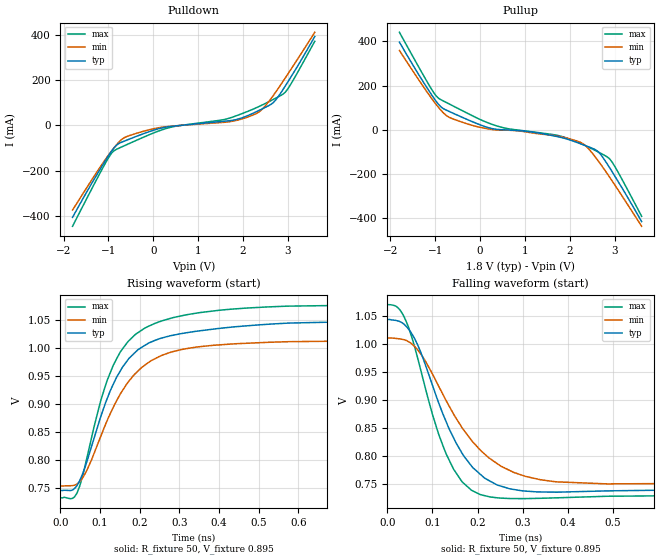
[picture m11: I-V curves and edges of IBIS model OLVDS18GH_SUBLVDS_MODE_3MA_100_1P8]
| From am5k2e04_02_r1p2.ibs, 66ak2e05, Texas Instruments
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|   Model Cell ilvds18gv
|   Model Cell olvds18gh
|   Model Cell OLVDS18GH_SUBLVDS_MODE_3MA_100_1P8
|OLVDS18GH_SUBLVDS_MODE_3MA_100_1P8
|olvds18gh.ibs [30Dec11 revision 1.0]
[Model]   OLVDS18GH_SUBLVDS_MODE_3MA_100_1P8
Model_type   Output
Polarity   Non-Inverting
Cref =  15.0001pF
Rref =  101.0000M
Vref =  0V
Vmeas =  1.08V
C_comp   1p   1p   1p
[Temperature Range]   25   125   -40
[Voltage Range]   1.8   1.62   1.98
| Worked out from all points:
|   slope of the pulldown table from 0 to 0.27 V, typ, clamps not added: 20.1 ohm
|   slope of the pullup table from 0 to 0.27 V, typ, clamps not added: 15.8 ohm
|   rising waveform, R_fixture 50, V_fixture 0.895: 20-80 % time 107ps typ, 116ps min, 96.1ps max; typ from 0.746 V to 1.04 V
|   falling waveform, R_fixture 50, V_fixture 0.895: 20-80 % time 90.7ps typ, 122ps min, 74.5ps max; typ from 1.04 V to 0.746 V
| Nom Voltages:
[Pulldown]
|   voltage   I(typ)   I(min)   I(max)
-1.8V     -406.9mA   -374.8mA   -446.6mA
-1.091V   -163.1mA   -157mA     -175.2mA
-872.7mV  -98.45mA   -98.29mA   -111.4mA
-654.5mV  -69.92mA   -54.94mA   -90.55mA
-54.55mV  -24.92mA   -17.11mA   -38.02mA
436.4mV   -3.309mA   -2.683mA   -5.734mA
1.745V    22.29mA    18.18mA    35.67mA
2.345V    65.48mA    58.17mA    83mA
2.673V    100.7mA    132mA      115.1mA
2.945V    175.7mA    211.4mA    148mA
3.109V    227.8mA    260.9mA    197.5mA
3.6V      394mA      412.8mA    372.8mA
[Pullup]
|   voltage   I(typ)   I(min)   I(max)
-1.8V     396.8mA    358.7mA    441.5mA
-1.145V   177.4mA    159.4mA    204.2mA
-927.3mV  114.3mA    100.5mA    142.1mA
-709.1mV  84.19mA    58.01mA    118.4mA
-109.1mV  30.59mA    15.72mA    56.53mA
490.9mV   -510.8uA   -2.408mA   10.05mA
1.745V    -32.6mA    -29.99mA   -26.98mA
2.291V    -68.08mA   -63.41mA   -67.31mA
2.618V    -97.7mA    -138mA     -99.79mA
2.891V    -174.1mA   -216.9mA   -133.5mA
3.109V    -246.4mA   -283.9mA   -205.6mA
3.6V      -417mA     -438.3mA   -393mA
[Ramp]
| variable   typ   min   max
dV/dt_f   9.252m/0.88253716n   5.154m/0.88425176n   11.244m/2.8474831n
dV/dt_r   4.506m/0.885501n   5.568m/3.3979628n   12.558m/4.1930989n
R_load = 50
[Rising Waveform]
R_fixture = 50
V_fixture = 0.895
V_fixture_min = 0.8825
V_fixture_max = 0.90115
|   time   V(typ)   V(min)   V(max)
0s        746.2mV    754.1mV    733.1mV
41.6ps    754.8mV    757.8mV    741.3mV
65.3ps    794.7mV    780.4mV    799.6mV
104ps     883mV      847.2mV    912.3mV
148.4ps   956.8mV    915.3mV    990.6mV
194.2ps   996.6mV    958.6mV    1.027V
238.6ps   1.014V     981.4mV    1.044V
339.3ps   1.03V      1.002V     1.062V
542.6ps   1.044V     1.011V     1.074V
1.262ns   1.045V     1.012V     1.072V
[Falling Waveform]
R_fixture = 50
V_fixture = 0.895
V_fixture_min = 0.8825
V_fixture_max = 0.90115
|   time   V(typ)   V(min)   V(max)
0s        1.045V     1.012V     1.071V
23.7ps    1.042V     1.01V      1.066V
45.8ps    1.029V     1.006V     1.033V
72.9ps    988.4mV    984.3mV    957.8mV
113.4ps   896.2mV    925.8mV    840.1mV
145.7ps   834.2mV    876.8mV    778.3mV
205.7ps   767.8mV    811.2mV    731.5mV
279.4ps   740.7mV    771.3mV    724.3mV
376.9ps   735.8mV    754.2mV    725.7mV
1.262ns   746.1mV    754.1mV    733.3mV
